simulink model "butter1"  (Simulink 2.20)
settings: Solver=VariableStepDiscrete  StartTime=0.0  StopTime=20.0  RelTol=1e-3  AbsTol=1e-6
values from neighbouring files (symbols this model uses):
  a = input('Inserisci il dato da graficare [1=PIDNL 2=PD 3=PID]: ')    [grp.m]    (also in grp1.m = input('Inserisci il dato da graficare [1..3]'))
undefined symbols (not defined in the file or in its folder): b, d1, n1

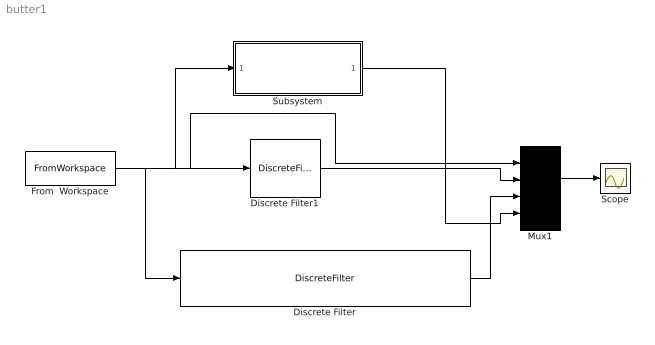
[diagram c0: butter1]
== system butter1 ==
  Discrete Filter : DiscreteFilter  Numerator="[0.00002411    0.00007232    0.00007232    0.00002411]"  Denominator="[1.0000   -2.8822    2.7713   -0.8889]"  SampleTime=0.033
  Discrete Filter1 : DiscreteFilter  Numerator=n1  Denominator=d1  SampleTime=.033
  From  Workspace : FromWorkspace  VariableName=[out(:,1),out(:,12)]
  Mux1 : Mux  Inputs=4
  Scope : Scope
  Subsystem : Subsystem  mask(Filtro di Butterworth){ordine=3, freq=0.6/16}
      mask prompts: ordine "Ordine del filtro"; freq "Parametro K per ricavare la Freq. di taglio Ft"
      mask help: Attenzione! Considerare il parametro Fc come la frequanza di campionamento del segnale di ingresso, per cui la frequanza di taglio diviene Ft=K*Fc;
      mask init:
      | [b,a]=butter(ordine,freq);
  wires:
  Mux1/1 -> Scope/1
  Discrete Filter/1 -> Mux1/3
  From  Workspace/1 -> Discrete Filter1/1, Mux1/1, Discrete Filter/1, Subsystem/1(In1)
  Discrete Filter1/1 -> Mux1/2
  Subsystem/1(Out1) -> Mux1/4

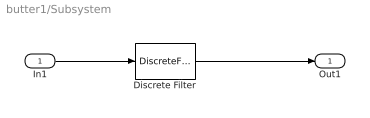
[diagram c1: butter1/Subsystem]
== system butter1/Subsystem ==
  In1 : Inport  Port=1  PortWidth=-1  SampleTime=-1
  Discrete Filter : DiscreteFilter  Numerator=b  Denominator=a  SampleTime=.033
  Out1 : Outport  Port=1
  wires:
  In1/1 -> Discrete Filter/1
  Discrete Filter/1 -> Out1/1
